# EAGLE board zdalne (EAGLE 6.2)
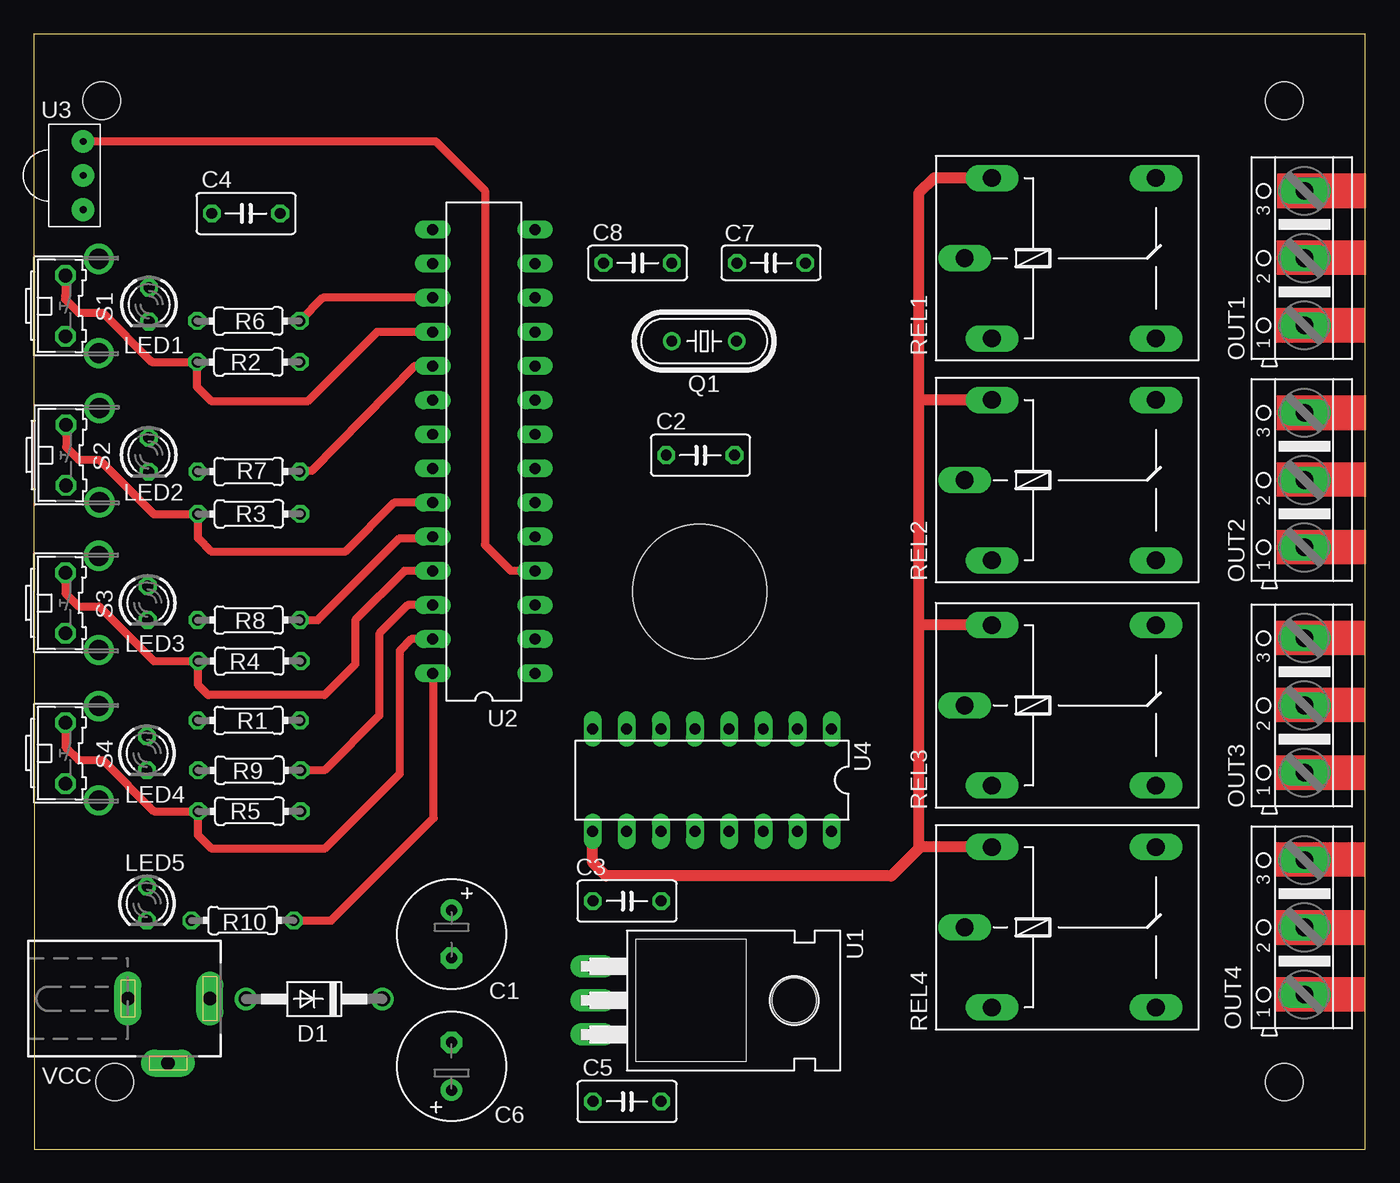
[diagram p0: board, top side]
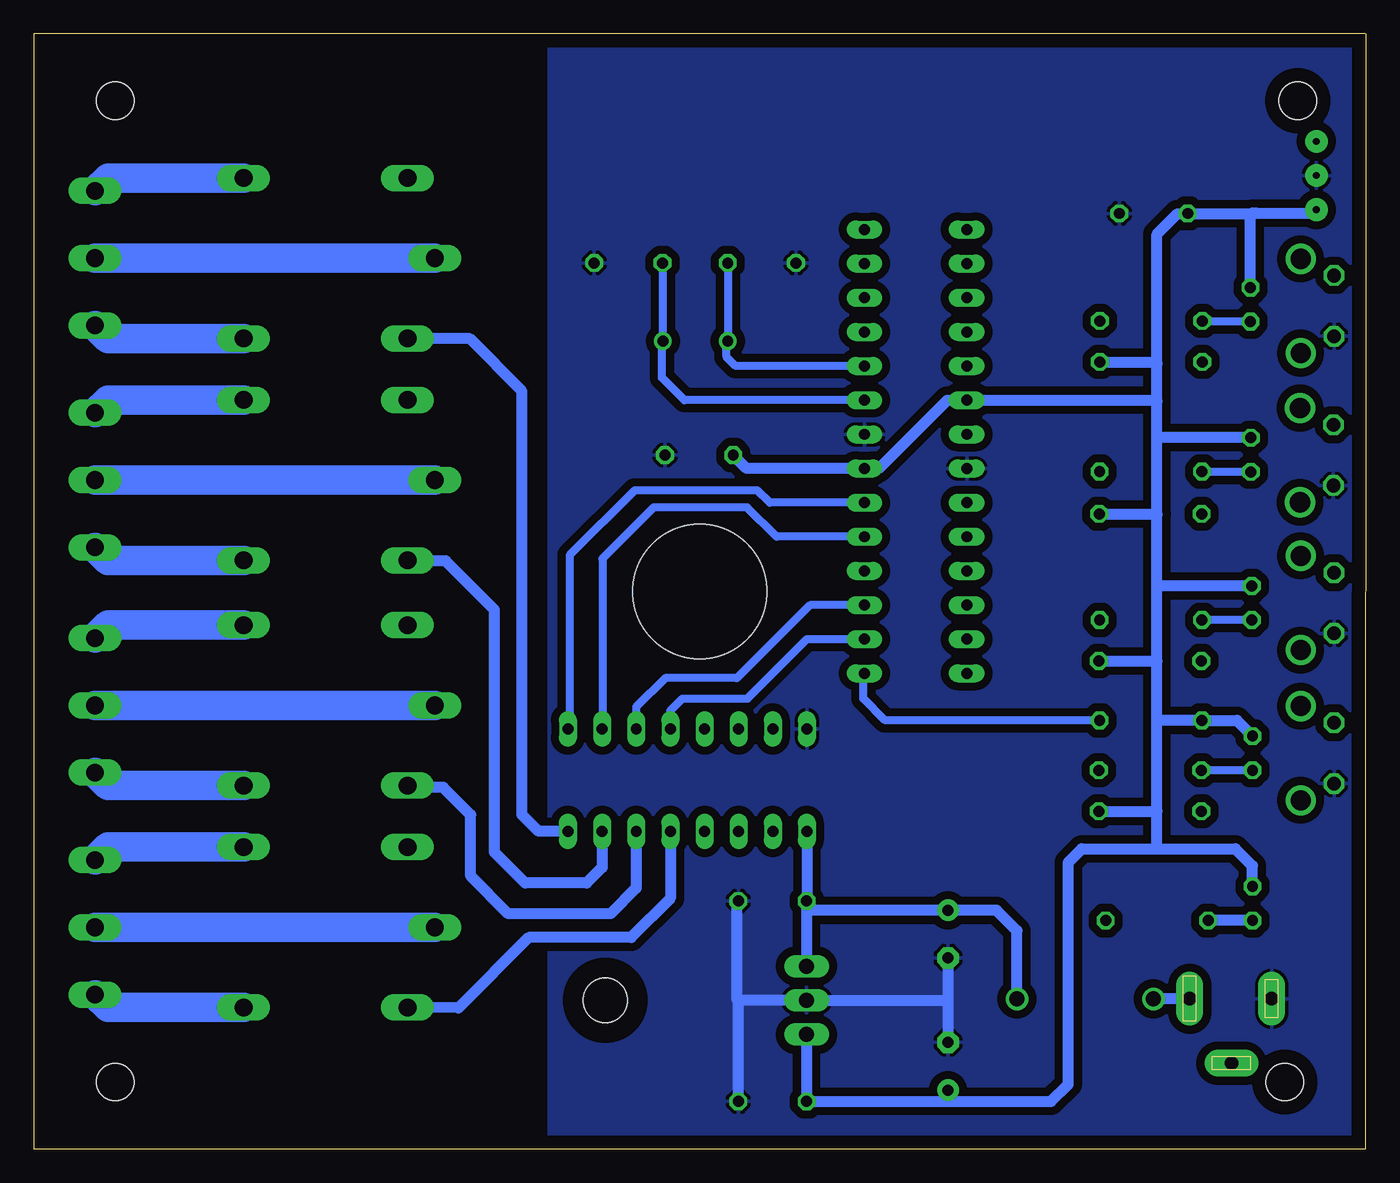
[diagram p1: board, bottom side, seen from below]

Size 99.05 x 83 mm. Coordinates in mm from the lower left corner, seen from the top.
Outline: 0,83 0.05,0 99.05,0 99.05,83 0.05,83
Copper layers (1*16): Top 0.035mm / dielectric 1.5mm / Bottom 0.035mm
Design rules: minimum track width 10mil, minimum drill 24mil, track to track 8mil, track to pad 8mil, pad to pad 8mil, via to via 8mil, smd to smd 8mil, copper to edge 40mil, drill to drill 8mil, minimum pad ring 10mil, minimum via ring 8mil, stop-mask expansion 4mil, vias tented up to drill 0mil, thermal gap 10mil
Holes 2.8 mm at 5.05,78 93.05,78 6.05,5 93.05,5
Holes 10 mm at 49.55,41.5

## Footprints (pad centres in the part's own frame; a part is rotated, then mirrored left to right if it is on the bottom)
E3,5-8 = drill 0.813 pad 1.6: + -1.778,0 | drill 0.813 pad 1.6 octagon: - 1.778,0
C050-030X075 = drill 0.813 octagon: 1 -2.54,0; 2 2.54,0
C050-025X075 = drill 0.813 octagon: 1 -2.54,0; 2 2.54,0
DO41-10 = drill 1.118: A 5.08,0; C -5.08,0
LED3MM = drill 0.813 octagon: A -1.27,0; K 1.27,0
AK500/3 = drill 1.321 long: 1 -5.004,0; 2 0,0; 3 5.004,0
HC49/S = drill 0.813: 1 -2.413,0; 2 2.413,0
0204/7 = drill 0.813 octagon: 1 -3.81,0; 2 3.81,0
G5LE = drill 1.321 long: 1 -7.493,-5.969; 2 -7.493,5.969; O 4.699,5.969; P -9.525,0; S 4.699,-5.969
B3F-31XX = drill 1.016 octagon: 1 -2.261,-1.245; 2 2.261,-1.245 | drill 1.499 pad 2.159: 3 -3.505,1.245; 4 3.505,1.245
TO220H = drill 1.118 long: 1 -2.54,-10.16; 2 0,-10.16; 3 2.54,-10.16 | hole 3.302: 0,4.826
DIL28-3 = drill 0.813 long: 1 -16.51,-3.81; 2 -13.97,-3.81; 3 -11.43,-3.81; 4 -8.89,-3.81; 5 -6.35,-3.81; 6 -3.81,-3.81; 7 -1.27,-3.81; 8 1.27,-3.81; 9 3.81,-3.81; 10 6.35,-3.81; 11 8.89,-3.81; 12 11.43,-3.81; 13 13.97,-3.81; 14 16.51,-3.81; 15 16.51,3.81; 16 13.97,3.81; 17 11.43,3.81; 18 8.89,3.81; 19 6.35,3.81; 20 3.81,3.81; 21 1.27,3.81; 22 -1.27,3.81; 23 -3.81,3.81; 24 -6.35,3.81; 25 -8.89,3.81; 26 -11.43,3.81; 27 -13.97,3.81; 28 -16.51,3.81
SFH5111 = drill 0.5 pad 1.676: GND 0,2.54; OUT 0,0; VCC 0,5.08
DIL16 = drill 0.813 long: 1 -8.89,-3.81; 2 -6.35,-3.81; 3 -3.81,-3.81; 4 -1.27,-3.81; 5 1.27,-3.81; 6 3.81,-3.81; 7 6.35,-3.81; 8 8.89,-3.81; 9 8.89,3.81; 10 6.35,3.81; 11 3.81,3.81; 12 1.27,3.81; 13 -1.27,3.81; 14 -3.81,3.81; 15 -6.35,3.81; 16 -8.89,3.81
DCJ0303 = drill 1 pad 2 long: 1 0,3.1; 2 4.8,0; 3 0,-3

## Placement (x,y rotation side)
C1  1000uF  [E3,5-8]  31.09,16 270 top
C2  100nF  [C050-030X075]  49.61,51.64 0 top
C3  100nF  [C050-030X075]  44.15,18.47 0 top
C4  100nF  [C050-030X075]  15.8,69.62 0 top
C5  100nF  [C050-030X075]  44.15,3.56 0 top
C6  470  [E3,5-8]  31.09,6.17 90 top
C7  22pF  [C050-025X075]  54.86,65.94 180 top
C8  22pF  [C050-025X075]  44.93,65.94 0 top
D1  1N4004  [DO41-10]  20.88,11.18 180 top
LED1  [LED3MM]  8.59,62.84 270 top
LED2  [LED3MM]  8.56,51.66 270 top
LED3  [LED3MM]  8.48,40.64 270 top
LED4  [LED3MM]  8.43,29.46 270 top
LED5  [LED3MM]  8.43,18.29 270 top
OUT1  [AK500/3]  94.54,66.29 90 top
OUT2  [AK500/3]  94.54,49.78 90 top
OUT3  [AK500/3]  94.54,33.02 90 top
OUT4  [AK500/3]  94.54,16.51 90 top
Q1  16MHz  [HC49/S]  49.89,60.12 0 top
R1  10k  [0204/7]  16,31.9 180 top
R2  10k  [0204/7]  15.98,58.57 0 top
R3  10k  [0204/7]  16.03,47.27 0 top
R4  10k  [0204/7]  16.05,36.32 0 top
R5  10k  [0204/7]  16.05,25.15 0 top
R6  1k  [0204/7]  15.98,61.62 0 top
R7  1k  [0204/7]  16,50.42 0 top
R8  1k  [0204/7]  16,39.37 180 top
R9  1k  [0204/7]  16.05,28.19 180 top
R10  1k  [0204/7]  15.54,17.02 180 top
REL1  G5LE  [G5LE]  78.79,66.29 0 top
REL2  G5LE  [G5LE]  78.79,49.78 0 top
REL3  G5LE  [G5LE]  78.79,33.02 0 top
REL4  G5LE  [G5LE]  78.79,16.51 0 top
S1  [B3F-31XX]  3.61,62.74 270 top
S2  [B3F-31XX]  3.66,51.64 270 top
S3  [B3F-31XX]  3.61,40.64 270 top
S4  [B3F-31XX]  3.61,29.46 270 top
U1  7805T  [TO220H]  51.77,11.07 270 top
U2  MEGA8-P  [DIL28-3]  33.5,51.92 90 top
U3  [SFH5111]  3.68,74.98 180 top
U4  ULN2003AN  [DIL16]  50.47,27.46 180 top
VCC  [DCJ0303]  10.01,11.2 270 top

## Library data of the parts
C1-C8 R1-R10 = rcl
D1 = diode
LED1-LED5 = led
OUT1-OUT4 = con-ptr500; OC_FARNELL: unknown; OC_NEWARK: unknown
Q1 = crystal; OC_FARNELL: 1667008; OC_NEWARK: unknown
REL1-REL4 = relay; OC_FARNELL: unknown; OC_NEWARK: unknown
S1-S4 = switch-omron; MPN: B3F-3100; OC_FARNELL: 959704; OC_NEWARK: 36M3582
U1 = linear
U2 = atmel; OC_FARNELL: unknown; OC_NEWARK: unknown
U3 = sfh511x
U4 = uln-udn
VCC = con-jack; OC_FARNELL: unknown; OC_NEWARK: unknown

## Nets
+5V: C2.1 C4.1 C5.1 C6.+ LED1.A LED2.A LED3.A LED4.A LED5.A R1.2 R2.2 R3.2 R4.2 R5.2 U1.3 U2.7 U2.20 U3.VCC
+12V: C1.+ C3.1 D1.C REL1.2 REL2.2 REL3.2 REL4.2 U1.1 U4.9
GND: C1.- C2.2 C3.2 C4.2 C5.2 C6.- C7.1 C8.1 S1.2 S2.2 S3.2 S4.2 U1.2 U2.8 U2.22 U3.GND U4.8 VCC.3
IR: U2.4 U3.OUT
LED1: R6.2 U2.17
LED2: R7.2 U2.19
LED3: R8.1 U2.24
LED4: R9.1 U2.26
LED5: R10.1 U2.28
N$1: LED4.K R9.2
N$2: LED5.K R10.2
N$8: REL1.1 U4.16
N$9: REL2.1 U4.15
N$10: REL3.1 U4.14
N$11: REL4.1 U4.13
N$13: LED1.K R6.1
N$14: R1.1 U2.1
N$15: C7.2 Q1.2 U2.9
N$16: OUT1.2 REL1.P
N$17: LED3.K R8.2
N$18: OUT3.2 REL3.P
N$19: OUT4.2 REL4.P
N$20: LED2.K R7.1
N$21: C8.2 Q1.1 U2.10
N$22: OUT2.2 REL2.P
N$23: OUT1.3 REL1.O
N$24: OUT1.1 REL1.S
N$25: D1.A VCC.1
N$26: OUT2.3 REL2.O
N$28: OUT2.1 REL2.S
N$29: OUT3.3 REL3.O
N$30: OUT3.1 REL3.S
N$32: OUT4.3 REL4.O
N$33: OUT4.1 REL4.S
P1: U2.6 U4.1
P2: U2.5 U4.2
P3: U2.3 U4.3
P4: U2.2 U4.4
S1: R2.1 S1.1 U2.18
S2: R3.1 S2.1 U2.23
S3: R4.1 S3.1 U2.25
S4: R5.1 S4.1 U2.27

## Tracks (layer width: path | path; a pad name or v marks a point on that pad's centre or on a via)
+5V
  Bottom 0.813: U1.3 C5.1 31.04,3.56 | 31.04,3.56 23.42,3.56 22.15,4.83 22.15,21.34 21.13,22.35 15.54,22.35 | C6.+ 31.09,3.61 31.04,3.56 | 15.54,22.35 15.54,25.15 | 15.54,25.15 15.54,31.75 | 15.54,31.75 15.54,36.32 | 15.54,36.32 15.54,42.16 | 15.54,42.16 15.54,47.24 | 15.54,47.24 15.54,53.09 | 15.54,53.09 15.54,55.63 | 15.54,55.63 15.54,58.42 | 15.54,58.42 15.54,68.07 14.02,69.6 13.28,69.6 C4.1 8.2,69.62 8.18,69.65 | 8.18,69.65 8.43,69.65 8.58,69.49 LED1.A | 8.18,69.65 3.94,69.65 U3.VCC | 15.6,58.62 15.54,58.42 | LED2.A 15.39,52.93 15.54,53.09 | 15.52,47.22 15.54,47.24 | LED3.A 15.29,41.91 15.54,42.16 | 15.54,55.63 15.65,55.73 U2.20 31.14,55.73 36.22,50.65 U2.7 46.08,50.65 C2.1 | LED5.A 8.43,21.08 9.7,22.35 15.54,22.35 | R5.2 15.54,25.15 | R4.2 15.54,36.32 | R3.2 15.57,47.27 15.54,47.24 | R2.2 15.7,58.57 15.54,58.42 | 15.54,31.75 15.39,31.9 R1.2 9.6,31.9 LED4.A
+12V
  Top 0.813: REL1.2 66.98,72.26 65.84,71.12 65.84,55.63 | 65.84,55.63 65.84,38.86 | 65.84,38.86 65.84,22.61 | 65.84,22.61 65.84,22.35 63.8,20.32 42.6,20.32 41.58,21.34 U4.9 | REL4.2 65.96,22.48 65.84,22.61 | REL3.2 65.96,38.99 65.84,38.86 | REL2.2 65.96,55.75 65.84,55.63
  Bottom 0.813: D1.C 25.96,16.26 27.48,17.78 C1.+ 41.45,17.78 41.45,18.31 C3.1 | C3.1 U1.1 | U4.9 41.58,18.57 C3.1
GND
  Bottom 0.813: C1.- 31.09,10.92 | 31.09,10.92 C6.- | 31.09,10.92 31.24,11.07 U1.2 46.53,11.07 | 46.53,11.07 46.68,11.07 46.79,11.18 46.79,18.36 C3.2 | C5.2 46.68,10.92 46.53,11.07
  pour Bottom (isolate 0.61): -1.73,84.33 60.76,84.33 60.76,-1.52 -1.47,-1.52
IR
  Top 0.61: U3.OUT 29.92,74.98 33.58,71.32 33.58,44.96 35.48,43.05 37.29,43.05 U2.4
LED1
  Top 0.61: U2.17 21.51,63.35 R6.2
LED2
  Top 0.61: U2.19 28.35,58.27 20.7,50.47 19.86,50.47 R7.2
LED3
  Top 0.61: R8.1 21.13,39.37 27.23,45.47 29.59,45.47 U2.24
LED4
  Top 0.61: U2.26 27.84,40.49 25.7,38.35 25.7,32.26 21.64,28.19 R9.1
LED5
  Top 0.61: R10.1 22.15,17.02 29.77,24.64 29.77,35.33 U2.28
N$1
  Bottom 0.61: LED4.K R9.2
N$2
  Bottom 0.813: LED5.K R10.2
N$8
  Bottom 0.813: U4.16 61.54,23.65 62.79,24.89 62.79,56.39 66.65,60.3 70.97,60.3 REL1.1
N$9
  Bottom 0.813: U4.15 56.82,20.95 57.96,19.81 62.53,19.81 64.82,22.1 64.82,40.13 68.45,43.76 70.99,43.76 REL2.1
N$10
  Bottom 0.813: U4.14 54.28,19.43 56.18,17.53 63.8,17.53 66.6,20.32 66.6,24.89 68.63,26.92 71.17,26.92 REL3.1
N$11
  Bottom 0.813: U4.13 51.74,18.67 54.66,15.75 62.28,15.75 67.51,10.52 REL4.1
N$13
  Bottom 0.61: LED1.K 12.12,61.57 R6.1
N$14
  Bottom 0.61: R1.1 35.76,31.9 37.39,33.53 37.39,35.33 U2.1
N$15
  Bottom 0.61: U2.9 50.7,55.73 52.37,57.4 52.37,60.05 Q1.2 52.3,65.91 C7.2
N$16
  Bottom 2.184: OUT1.2 REL1.P
N$17
  Bottom 0.61: LED3.K R8.2
N$18
  Bottom 2.184: REL3.P OUT3.2
N$19
  Bottom 2.184: REL4.P OUT4.2
N$20
  Bottom 0.61: LED2.K 12.17,50.39 R7.1
N$21
  Bottom 0.61: C8.2 Q1.1 47.55,60.05 47.55,58.93 46.89,58.27 U2.10
N$22
  Bottom 2.184: OUT2.2 REL2.P
N$23
  Bottom 2.184: REL1.O 93.57,72.26 OUT1.3
N$24
  Bottom 2.184: REL1.S 93.57,60.33 OUT1.1
N$25
  Bottom 0.813: VCC.1 15.8,11.2 D1.A
N$26
  Bottom 2.184: REL2.O 93.57,55.75 OUT2.3
N$28
  Bottom 2.184: REL2.S 93.57,43.81 OUT2.1
N$29
  Bottom 2.184: REL3.O 93.57,38.99 OUT3.3
N$30
  Bottom 2.184: REL3.S 93.57,27.05 OUT3.1
N$32
  Bottom 2.184: REL4.O 93.57,22.48 OUT4.3
N$33
  Bottom 2.184: REL4.S 93.57,10.54 OUT4.1
P1
  Bottom 0.61: U2.6 44.35,48.11 45.26,49.02 54.41,49.02 59.23,44.2 59.23,31.39 U4.1
P2
  Bottom 0.61: U2.5 43.84,45.57 46.02,47.75 52.98,47.75 56.79,43.94 56.79,31.39 U4.2
P3
  Bottom 0.61: U2.3 41.35,40.49 46.79,35.05 52.12,35.05 54.28,32.92 U4.3 | U4.3 54.33,31.29 54.33,31.32 U4.3
P4
  Bottom 0.61: U4.4 51.74,32.64 50.85,33.53 46,33.53 41.58,37.95 U2.2
S1
  Top 0.61: S1.1 2.34,65 2.34,63.5 2.34,63.25 3.35,62.23 5.13,62.23 8.69,58.67 8.79,58.57 R2.1 12.17,56.72 13.26,55.63 20.37,55.63 25.55,60.81 U2.18
S2
  Top 0.61: S2.1 2.41,52.25 3.35,51.31 4.88,51.31 8.94,47.24 12.19,47.24 R3.1 12.24,47.24 12.24,45.47 13.26,44.45 23.16,44.45 26.82,48.11 U2.23
S3
  Top 0.61: S3.1 2.36,41.38 3.35,40.39 4.88,40.39 8.94,36.32 R4.1 12.24,34.54 13,33.78 21.64,33.78 23.93,36.07 23.93,39.37 27.58,43.03 U2.25
S4
  Top 0.61: S4.1 2.36,29.95 3.35,28.96 5.13,28.96 8.94,25.15 R5.1 12.24,23.37 13.26,22.35 21.64,22.35 27.23,27.94 27.23,37.08 28.09,37.95 U2.27
(copper drawn outside any net)
  shapes: Top area x13

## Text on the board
tNames: U3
